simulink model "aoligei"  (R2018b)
settings: Solver=VariableStepAuto  StartTime=0.0  StopTime=2  RelTol=1e-3
undefined symbols (not defined in the file): HP, RPM, V
libraries: powerlib x15, powerlib_meascontrol x1

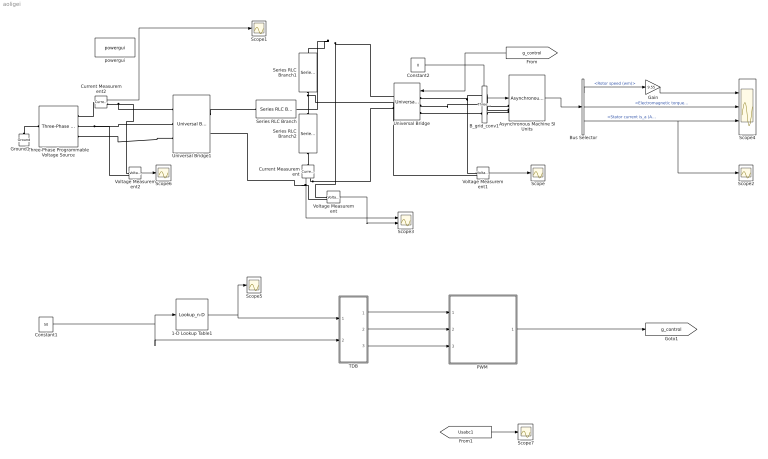
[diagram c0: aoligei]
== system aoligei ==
  1-D Lookup Table1 : Lookup_n-D  NumberOfTableDimensions=1  BreakpointsForDimension1=[0,50]  Table=[0,0.8]  InternalRulePriority=Speed  RndMeth=Simplest
  Asynchronous Machine SI Units : powerlib/Machines/Asynchronous Machine SI Units  RotorType=Squirrel-cage  PresetModel="15:  5.4 HP (4KW)   400 V  50Hz 1430 RPM"  MechanicalLoad=Torque Tm  ShowDetailedParameters=on  ReferenceFrame=Rotor  Units=SI  MeasurementBus=off  NominalParameters=[4000 400 50]  Stator=[1.405 0.005839]  Rotor=[1.395 0.005839]  Cage1=[0.4155 0.002066]  Cage2=[0.4168 0.0003495]  Lm=0.1722  Mechanical=[0.0131 0.002985 2]  PolePairs=2  InitialConditions=[1 0 0 0 0 0 0 0]  SimulateSaturation=off  Saturation=[14.03593122, 27.81365428, 53.79336849, 72.68890987, 97.98006896, 148.6815601, 215.7428561, 302.9841135, 428.7778367 ; 230, 322, 414, 460, 506, 552, 598, 644, 690]  LoadFlowParameters=1492000  TsPowergui=0  TsBlock=-1  IterativeModel=Trapezoidal non iterative  IterativeDiscreteModel=Trapezoidal non iterative  Pmec=1.492e+006
  B_grid_conv1 : powerlib/Measurements/Three-Phase V-I Measurement  VoltageMeasurement=phase-to-ground  SetLabelV=on  LabelV=Usabc1  Vpu=off  VpuLL=off  CurrentMeasurement=yes  SetLabelI=on  LabelI=Isabc1  Ipu=off  Pbase=Pnom  Vbase=Vnom  OutputType=Complex  PhasorSimulation=off  PSBequivalent=0
  Bus Selector : BusSelector  OutputSignals=Mechanical.Rotor speed (wm),Mechanical.Electromagnetic torque Te (N*m),Stator measurements.Stator current is_a (A)
  Constant1 : Constant  Value=50
  Constant2 : Constant  Value=0
  Current Measurement : powerlib/Measurements/Current Measurement  PhasorSimulation=off  OutputType=Complex  PSBequivalent=0
  Current Measurement2 : powerlib/Measurements/Current Measurement  PhasorSimulation=off  OutputType=Complex  PSBequivalent=0
  Gain : Gain  Gain=9.55
  Ground1 : powerlib/Elements/Ground  LConnTagsString=a
  "PWM " : Subsystem
  Scope{,1..2,5..7} (6 alike) : Scope
  Scope3 : Scope  NumInputPorts=2
  Scope4 : Scope  NumInputPorts=3
  Series RLC Branch : powerlib/Elements/Series RLC Branch  LConnTagsString=__new0  RConnTagsString=__new0  BranchType=R  Resistance=15  Inductance=1e-3  SetiL0=off  InitialCurrent=0  Capacitance=1e-6  Setx0=off  InitialVoltage=0  Measurements=None
  Series RLC Branch1 : powerlib/Elements/Series RLC Branch  LConnTagsString=__new0  RConnTagsString=__new0  BranchType=C  Resistance=1  Inductance=1e-3  SetiL0=off  InitialCurrent=0  Capacitance=4.4e-3  Setx0=off  InitialVoltage=0  Measurements=None
  Series RLC Branch2 : powerlib/Elements/Series RLC Branch  LConnTagsString=__new0  RConnTagsString=__new0  BranchType=C  Resistance=1  Inductance=1e-3  SetiL0=off  InitialCurrent=0  Capacitance=4.4e-3  Setx0=off  InitialVoltage=0  Measurements=None
  TDB : Subsystem
  Three-Phase Programmable Voltage Source : powerlib/Electrical Sources/Three-Phase Programmable Voltage Source  PositiveSequence=[380 0 50]  VariationEntity=None  VariationType=Table of time-amplitude pairs  VariationTypeAlt=Step  VariationStep=0.5  VariationRate=10  VariationMagnitude=0.3  VariationFrequency=2  VariationTiming=[1 2]  VariationPhaseA=off  Amplitudes=[1 0.2 1.0 ]  TimeValues=[0 1 1.5 ]  HarmonicGeneration=off  HarmonicA=[3 0.2 -25 0]  HarmonicB=[2 0.15 35 2]  Timing="[0.05  3]"  BusType=swing  Pref=0  Qref=0  Qmin=-inf  Qmax=inf
  Universal Bridge : powerlib/Power Electronics/Universal Bridge  Arms=3  SnubberResistance=1e5  SnubberCapacitance=inf  Device=IGBT / Diodes  Ron=1e-3  Lon=0  ForwardVoltages="[  0  0  ]"  ForwardVoltage=0  GTOparameters=[ 10e-6 , 20e-6 ]  IGBTparameters=[ 0 , 0 ]  Measurements=None  Measurements_2=None  converterType=Rectifier
  Universal Bridge1 : powerlib/Power Electronics/Universal Bridge  Arms=3  SnubberResistance=1e5  SnubberCapacitance=inf  Device=Diodes  Ron=1e-3  Lon=0  ForwardVoltages="[  0  0  ]"  ForwardVoltage=0  GTOparameters=[ 10e-6 , 20e-6 ]  IGBTparameters=[ 1e-6 , 2e-6 ]  Measurements=None  Measurements_2=None  converterType=Rectifier
  Voltage Measurement : powerlib/Measurements/Voltage Measurement  PhasorSimulation=off  OutputType=Complex  PSBequivalent=0
  Voltage Measurement1 : powerlib/Measurements/Voltage Measurement  PhasorSimulation=off  OutputType=Complex  PSBequivalent=0
  Voltage Measurement2 : powerlib/Measurements/Voltage Measurement  PhasorSimulation=off  OutputType=Complex  PSBequivalent=0
  powergui : powerlib/powergui  Priority=1  SimulationMode=Continuous  SampleTime=50e-6  frequency=60  Iterations=50  frequencyindice=50  Pbase=100e6  ErrMax=1e-4  UnitsV=kV  UnitsW=MW  buscounter=0  FunctionMessages=off  echomessages=off  EnableUseOfTLC=off  CurrentSourceSwitches=off  DisableSnubberDevices=off  DisableRonSwitches=off  DisableVfSwitches=off  DisplayEquations=off  SolverType=Tustin/Backward Euler (TBE)  Interpol=off  ExternalGateDelay=off  methode=off  Ts=100  x0status=blocks  SPID=on  SwTol=0  HookPort=off  RestoreLinks=warning  ResistiveCurrentMeasurement=off  Frange=[0:2:500]  Ylog=off  Xlog=on  ShowGrid=off  save=off  variable=ZData  structure=ScopeData  ZoomFFT=off  StartTime=0.0  cycles=2  DisplayStyle=1  fundamental=50  FreqAxis=off  MaxFrequency=1000  frequencyindicesteady=1  RmsSteady=1  display=off
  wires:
  Current Measurement/1 -> Scope3/1
  Constant2/1 -> Asynchronous Machine SI Units/1
  Asynchronous Machine SI Units/1 -> Bus Selector/1
  Bus Selector/1 -> Gain/1  "<Rotor speed (wm)>"
  Gain/1 -> Scope4/1
  Bus Selector/3 -> Scope2/1, Scope4/3  "<Stator current is_a (A)>"
  Voltage Measurement/1 -> Scope3/2
  Voltage Measurement1/1 -> Scope/1
  [g_control] -> Universal Bridge/1
  Bus Selector/2 -> Scope4/2  "<Electromagnetic torque Te (N*m)>"
  Current Measurement2/1 -> Scope1/1
  1-D Lookup Table1/1 -> Scope5/1, TDB/1(Voltage)
  TDB/1(ua) -> "PWM "/1(In1)
  TDB/2(ub) -> "PWM "/2(In2)
  TDB/3(uc) -> "PWM "/3(In3)
  "PWM "/1(Out) -> [g_control]
  Constant1/1 -> 1-D Lookup Table1/1, TDB/2(Frequency)
  Voltage Measurement2/1 -> Scope6/1
  [Usabc1] -> Scope7/1
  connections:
  Ground1/LConn1 -- Three-Phase Programmable Voltage Source/LConn1
  Series RLC Branch1/RConn1 -- Voltage Measurement1/LConn2 -- Series RLC Branch2/LConn1
  Current Measurement/LConn1 -- Series RLC Branch2/RConn1
  Voltage Measurement1/LConn1 -- B_grid_conv1/LConn1 -- Universal Bridge/LConn1
  Universal Bridge/RConn2 -- Universal Bridge1/RConn2 -- Voltage Measurement/LConn2 -- Current Measurement/RConn1
  Three-Phase Programmable Voltage Source/RConn2 -- Voltage Measurement2/LConn2 -- Universal Bridge1/LConn2
  Universal Bridge1/RConn1 -- Series RLC Branch/LConn1
  Voltage Measurement/LConn1 -- Series RLC Branch1/LConn1 -- Series RLC Branch/RConn1 -- Universal Bridge/RConn1
  Current Measurement2/LConn1 -- Three-Phase Programmable Voltage Source/RConn1
  Current Measurement2/RConn1 -- Voltage Measurement2/LConn1 -- Universal Bridge1/LConn1
  Three-Phase Programmable Voltage Source/RConn3 -- Universal Bridge1/LConn3
  B_grid_conv1/RConn1 -- Asynchronous Machine SI Units/LConn1
  B_grid_conv1/RConn2 -- Asynchronous Machine SI Units/LConn2
  B_grid_conv1/RConn3 -- Asynchronous Machine SI Units/LConn3
  B_grid_conv1/LConn2 -- Universal Bridge/LConn2
  B_grid_conv1/LConn3 -- Universal Bridge/LConn3

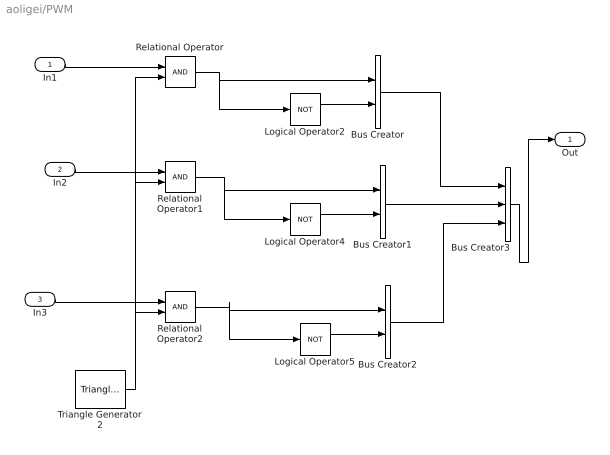
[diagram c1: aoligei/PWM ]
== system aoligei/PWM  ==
  In1 : Inport
  In2 : Inport  Port=2
  In3 : Inport  Port=3
  Bus Creator : BusCreator  Inputs=2
  Bus Creator1 : BusCreator  Inputs=2
  Bus Creator2 : BusCreator  Inputs=2
  Bus Creator3 : BusCreator  Inputs=3
  Logical Operator2 : Logic  Operator=NOT  AllPortsSameDT=off  OutDataTypeStr=boolean
  Logical Operator4 : Logic  Operator=NOT  AllPortsSameDT=off  OutDataTypeStr=boolean
  Logical Operator5 : Logic  Operator=NOT  AllPortsSameDT=off  OutDataTypeStr=boolean
  Relational Operator : RelationalOperator  OutDataTypeStr=boolean  RndMeth=Simplest
  Relational Operator1 : RelationalOperator  OutDataTypeStr=boolean  RndMeth=Simplest
  Relational Operator2 : RelationalOperator  OutDataTypeStr=boolean  RndMeth=Simplest
  Triangle Generator2 : powerlib_meascontrol/Pulse & Signal Generators/Triangle Generator  Freq=10e3  Phase=90  Ts=0
  Out : Outport
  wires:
  Relational Operator2/1 -> Bus Creator2/1, Logical Operator5/1
  In2/1 -> Relational Operator1/1
  Logical Operator4/1 -> Bus Creator1/2
  Bus Creator1/1 -> Bus Creator3/2
  Relational Operator1/1 -> Logical Operator4/1, Bus Creator1/1
  Bus Creator/1 -> Bus Creator3/1
  In3/1 -> Relational Operator2/1
  Bus Creator2/1 -> Bus Creator3/3
  Relational Operator/1 -> Logical Operator2/1, Bus Creator/1
  Triangle Generator2/1 -> Relational Operator/2, Relational Operator1/2, Relational Operator2/2
  Logical Operator2/1 -> Bus Creator/2
  Logical Operator5/1 -> Bus Creator2/2
  In1/1 -> Relational Operator/1
  Bus Creator3/1 -> Out/1

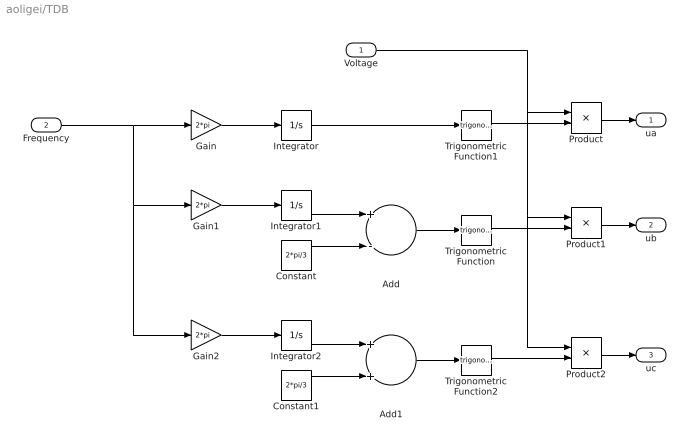
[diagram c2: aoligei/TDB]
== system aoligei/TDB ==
  Voltage : Inport
  Frequency : Inport  Port=2
  Add : Sum  Inputs=+-
  Add1 : Sum
  Constant : Constant  Value=2*pi/3
  Constant1 : Constant  Value=2*pi/3
  Gain : Gain  Gain=2*pi
  Gain1 : Gain  Gain=2*pi
  Gain2 : Gain  Gain=2*pi
  Integrator : Integrator
  Integrator1 : Integrator
  Integrator2 : Integrator
  Product : Product
  Product1 : Product
  Product2 : Product
  Trigonometric Function : Trigonometry
  Trigonometric Function1 : Trigonometry
  Trigonometric Function2 : Trigonometry
  ua : Outport
  ub : Outport  Port=2
  uc : Outport  Port=3
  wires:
  Integrator2/1 -> Add1/1
  Integrator1/1 -> Add/1
  Constant1/1 -> Add1/2
  Constant/1 -> Add/2
  Voltage/1 -> Product1/1, Product2/1, Product/1
  Frequency/1 -> Gain1/1, Gain2/1, Gain/1
  Trigonometric Function2/1 -> Product2/2
  Gain2/1 -> Integrator2/1
  Trigonometric Function1/1 -> Product/2
  Add1/1 -> Trigonometric Function2/1
  Integrator/1 -> Trigonometric Function1/1
  Gain/1 -> Integrator/1
  Gain1/1 -> Integrator1/1
  Add/1 -> Trigonometric Function/1
  Trigonometric Function/1 -> Product1/2
  Product2/1 -> uc/1
  Product1/1 -> ub/1
  Product/1 -> ua/1
